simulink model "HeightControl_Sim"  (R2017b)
settings: Solver=ode4  StartTime=0.0  StopTime=2  FixedStep=0.001  RelTol=1e-3
InitFcn:
  | Init_control;
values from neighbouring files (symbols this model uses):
  DEG2RAD = 0.0174533    [Init_control.m]
  Kd_PITCH_AngleRate = 0.001    [Init_control.m]
  Kd_ROLL_AngleRate = 0.001    [Init_control.m]
  Kd_YAW_AngleRate = 0.00    (= 0)    [Init_control.m]
  Ki_PITCH_AngleRate = 0.02    [Init_control.m]
  Ki_ROLL_AngleRate = 0.02    [Init_control.m]
  Ki_YAW_AngleRate = 0.001    [Init_control.m]
  Kp_PITCH_ANGLE = 6.5    [Init_control.m]
  Kp_PITCH_AngleRate = 0.1    [Init_control.m]
  Kp_ROLL_ANGLE = 6.5    [Init_control.m]
  Kp_ROLL_AngleRate = 0.1    [Init_control.m]
  Kp_YAW_AngleRate = 0.3    [Init_control.m]
  Kpxp = 1.0    (= 1)    [Init_control.m]
  Kpyp = 1.0    (= 1)    [Init_control.m]
  Kpzp = 4.0    (= 4)    [Init_control.m]
  Kvxd = 0.01    [Init_control.m]
  Kvxi = 0.4    [Init_control.m]
  Kvxp = 2.5    [Init_control.m]
  Kvyd = 0.01    [Init_control.m]
  Kvyi = 0.4    [Init_control.m]
  Kvyp = 2.5    [Init_control.m]
  Kvzd = 0.005    [Init_control.m]
  Kvzi = 0.01    [Init_control.m]
  Kvzp = 0.45    [Init_control.m]
  MAX_CONTROL_ANGLE_PITCH = 35    [Init_control.m]
  MAX_CONTROL_ANGLE_RATE_PITCH = 220    [Init_control.m]
  MAX_CONTROL_ANGLE_RATE_ROLL = 220    [Init_control.m]
  MAX_CONTROL_ANGLE_RATE_Y = 200    [Init_control.m]
  MAX_CONTROL_ANGLE_ROLL = 35    [Init_control.m]
  MAX_CONTROL_VELOCITY_XY = 5    [Init_control.m]
  MAX_CONTROL_VELOCITY_Z = 3    [Init_control.m]
  ModelInit_AngEuler = [0, 0, 0]    [Init_control.m]    (also in Init.m)
  ModelInit_PosE = [0, 0, -100]    [Init_control.m]    (also in Init.m = [0, 0, 0])
  ModelInit_Rads = 0    [Init_control.m]    (also in Init.m)
  ModelInit_RateB = [0, 0, 0]    [Init_control.m]    (also in Init.m)
  ModelInit_VelB = [0, 0, 0]    [Init_control.m]    (also in Init.m)
  ModelParam_envGravityAcc = 9.8    [Init.m]
  ModelParam_motorCr = 1148    [Init.m]
  ModelParam_motorJm = 0.0001287    [Init.m]
  ModelParam_motorT = 0.02    [Init.m]
  ModelParam_motorWb = -141.4    [Init.m]
  ModelParam_rotorCm = 1.779e-07    [Init.m]
  ModelParam_rotorCt = 1.105e-05    [Init.m]
  ModelParam_uavCCm = [0.0035 0.0039 0.0034]    [Init.m]
  ModelParam_uavCd = 0.055    [Init.m]
  ModelParam_uavJ = [ModelParam_uavJxx, 0, 0;     0, ModelParam_uavJyy, 0;     0, 0, ModelParam_uavJzz]    [Init.m]
  ModelParam_uavMass = 1.4    [Init.m]
  ModelParam_uavR = 0.225    [Init.m]
  Saturation_I_ah = 3.43    [Init_control.m]
  Saturation_I_az = 5    [Init_control.m]
  Saturation_I_RP_Max = 0.3    [Init_control.m]
  Saturation_I_RP_Min = -0.3    [Init_control.m]
  Saturation_I_Y_Max = 0.2    [Init_control.m]
  Saturation_I_Y_Min = -0.2    [Init_control.m]
  THR_HOVER = 0.609    [Init_control.m]
undefined symbols (not defined in the file or in its folder): Column, D, DiscIntNeverNeededParam, earthRadius, Receive, Send, vector
libraries: simulink x8, aerolibfltsims x3, sharedutil x2, aerolibanimutils x1
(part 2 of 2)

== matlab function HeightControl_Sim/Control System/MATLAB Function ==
function [vx_d, vy_d, vz_d, x_d, y_d, z_d]  = fcn(vzd, x, y, z, vx, vy, vz)
%Function description:
%  Implementation of altitude control logic. When the desired velocity
%  along OeZe(vzd) is < 0.001, and the current velocity along OeZe(vz) is
%  <6 m/s, the altitude hold is activated, and the desired altitude is the
%  altitude at the moment when the above condition is satisfied. The height
%  loop and the velocity loop act simultaneously. When the condition is not
%  satisfied, only altitude velocity feedback works for the altitude
%  controller.
%Input:
%  vzd: the desired velocity along OeZe
%  x, y, z: current position
%  vx, vy, vz: current velocity
%Output:
%  vx_d, vy_d, vz_d, x_d, y_d, z_d: desired velocity and position to
%  position controller
persistent z1;
if isempty(z1)
    z1= z;
end
persistent hold_z_flag;
if isempty(hold_z_flag)
    hold_z_flag = 0;
end

if abs(vzd) < 0.001 && abs(vz) < 6
    hold_z = 1;
else
    hold_z = 0;
    hold_z_flag = 0;
end

% throttle in the middle position, hold the altitude
if (hold_z > 0.5) && (hold_z_flag < 0.5)
    z1 = z;
    hold_z_flag = 1;
end
%The throttle control stick deviates from the middle position, i.e., out
% of the dead zone range, the desired altitude is changed to the current
% altitude. 
if hold_z < 0.5
    z1 = z;
    hold_z_flag = 0;
end
vx_d = vx; vy_d = vy; vz_d = vzd;

x_d = x;
y_d = y;
z_d = z1;

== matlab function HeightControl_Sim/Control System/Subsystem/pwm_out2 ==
function [M1, M2, M3, M4] = motor_mixer(Roll, Pitch, Yaw, Thrust)
%Function description:
%  Control allocation. The quadrotor type is X-configuration,
%  and the airframe is as follows:
%3↓   1↑
 %  \ /
 %  / \
 %2↑   4↓
%Input：
%  Roll, Pitch, Yaw: attitude controller output.
%  Thrust

idle_PWM = 1000;
scale = 1000;

M1 = (Thrust - Roll + Pitch + Yaw) * scale + idle_PWM;
M2 = (Thrust + Roll - Pitch + Yaw) * scale + idle_PWM;
M3 = (Thrust + Roll + Pitch - Yaw) * scale + idle_PWM;
M4 = (Thrust - Roll - Pitch - Yaw) * scale + idle_PWM;

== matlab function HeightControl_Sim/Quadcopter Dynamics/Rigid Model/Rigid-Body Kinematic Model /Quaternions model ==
function qdot = fcn(pqr, q)
%Function description:
%  Quaternions model
qdot = 0.5*[0, -pqr(1), -pqr(2), -pqr(3); pqr(1), 0, pqr(3), -pqr(2); pqr(2), -pqr(3), 0, pqr(1); pqr(3), pqr(2), -pqr(1), 0]*q;

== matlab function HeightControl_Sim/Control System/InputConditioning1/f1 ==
function y = thr_curve(in, hover)
%Function description:
%  throttle curve. When the throttle is in the middle position, the output
%  is hovering throttle value.
%Input:
%  in: normalized throttle, range from 0 to 1
%  hover: hovering throttle value
%Output:
%  y: processed throttle value
if in < 0.5
	y=2 * in * hover;
else
	y=hover + 2 * (in - 0.5) * (1.0 - hover);
end
